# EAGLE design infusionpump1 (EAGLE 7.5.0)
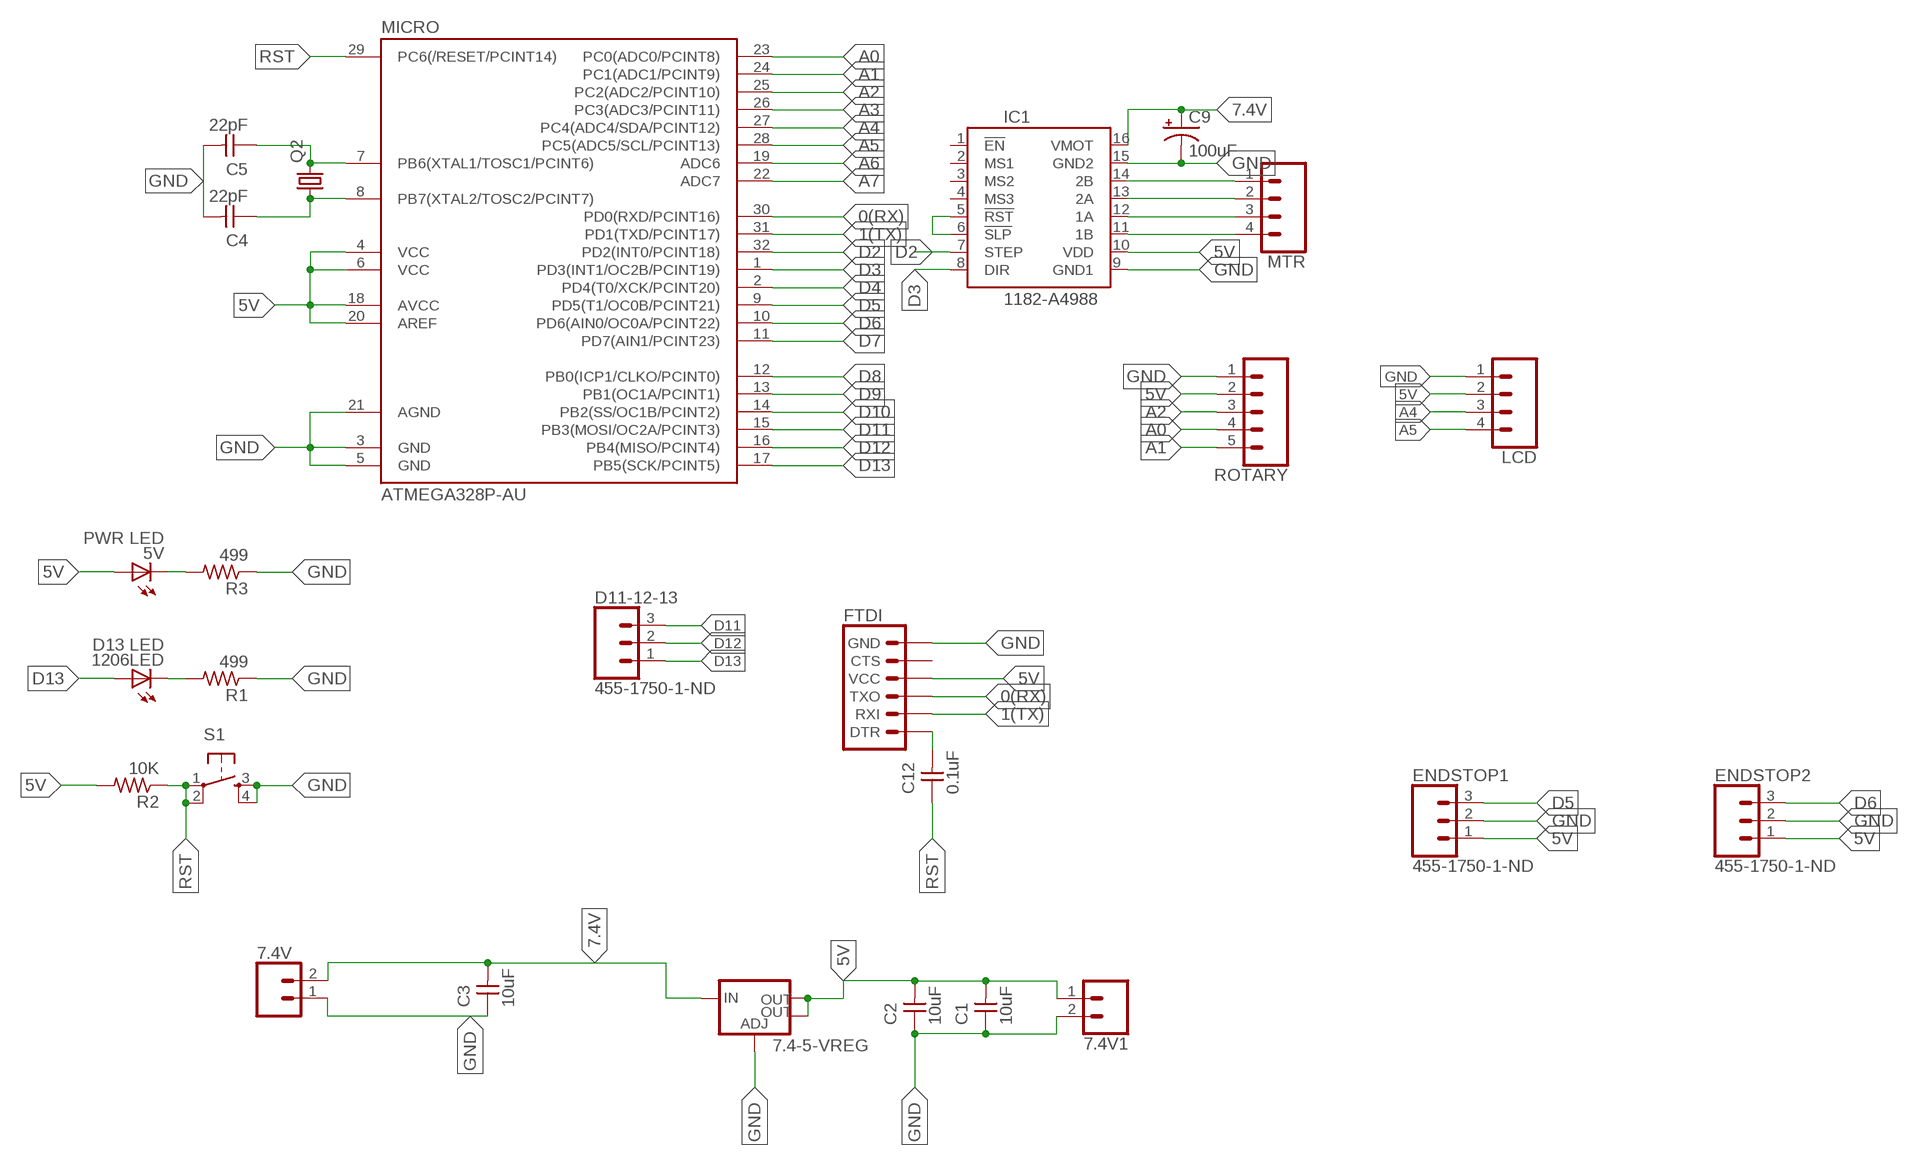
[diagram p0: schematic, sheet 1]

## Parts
5V  PWR LED  LEDFAB1206  [LED1206FAB]
7.4-5-VREG  V_REG_LM1117SOT223  [SOT223]
7.4V  CONN_02LOCK  [1X02_LOCK]
7.4V1  CONN_02LOCK  [1X02_LOCK]
1206LED  D13 LED  LEDFAB1206  [LED1206FAB]
C1  10uF  CAP-UNPOLARIZEDFAB  [C1206FAB]
C2  10uF  CAP-UNPOLARIZEDFAB  [C1206FAB]
C3  10uF  CAP-UNPOLARIZEDFAB  [C1206FAB]
C4  22pF  CAP-UNPOLARIZEDFAB  [C1206FAB]
C5  22pF  CAP-UNPOLARIZEDFAB  [C1206FAB]
C9  100uF  1000UF-RADIAL-5MM-25V-20%  [CPOL-RADIAL-5MM-10MM]
C12  0.1uF  CAP-UNPOLARIZEDFAB  [C1206FAB]
D11-12-13  455-1750-1-ND  CONN_03  [1X03]
ENDSTOP1  455-1750-1-ND  CONN_03  [1X03]
ENDSTOP2  455-1750-1-ND  CONN_03  [1X03]
FTDI  6_PIN_SERIAL_TARGET_SILK  [1X06]
IC1  1182-A4988  [A4988]
LCD  CONN_04  [1X04]
MICRO  ATMEGA328P-AU  ATMEGA48/88/168-AU  [TQFP32-08]
MTR  CONN_04  [1X04]
Q2  CRYSTALHC49U70  [HC49U70]
R1  499  RES-US1206FAB  [R1206FAB]
R2  10K  RES-US1206FAB  [R1206FAB]
R3  499  RES-US1206FAB  [R1206FAB]
ROTARY  CONN_05  [1X05]
S1  6MM_SWITCH6MM_SWITCH  [6MM_SWITCH]

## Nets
0(RX): FTDI.3(TXO) MICRO.30(PD0(RXD/PCINT16))
1(TX): FTDI.2(RXI) MICRO.31(PD1(TXD/PCINT17))
5V: 5V.1(A) 7.4-5-VREG.2(OUT) 7.4-5-VREG.4(OUT) 7.4V1.1 C1.2 C2.2 ENDSTOP1.1 ENDSTOP2.1 FTDI.4(VCC) IC1.10(VDD) LCD.2 MICRO.4(VCC) MICRO.6(VCC) MICRO.18(AVCC) MICRO.20(AREF) R2.2 ROTARY.2
7.4V: 7.4-5-VREG.3(IN) 7.4V.2 C3.2 C9.+ IC1.16(VMOT)
A0: MICRO.23(PC0(ADC0/PCINT8)) ROTARY.4
A1: MICRO.24(PC1(ADC1/PCINT9)) ROTARY.5
A2: MICRO.25(PC2(ADC2/PCINT10)) ROTARY.3
A3: MICRO.26(PC3(ADC3/PCINT11))
A4: LCD.3 MICRO.27(PC4(ADC4/SDA/PCINT12))
A5: LCD.4 MICRO.28(PC5(ADC5/SCL/PCINT13))
A6: MICRO.19(ADC6)
A7: MICRO.22(ADC7)
D2: IC1.7(STEP) MICRO.32(PD2(INT0/PCINT18))
D3: IC1.8(DIR) MICRO.1(PD3(INT1/OC2B/PCINT19))
D4: MICRO.2(PD4(T0/XCK/PCINT20))
D5: ENDSTOP1.3 MICRO.9(PD5(T1/OC0B/PCINT21))
D6: ENDSTOP2.3 MICRO.10(PD6(AIN0/OC0A/PCINT22))
D7: MICRO.11(PD7(AIN1/PCINT23))
D8: MICRO.12(PB0(ICP1/CLKO/PCINT0))
D9: MICRO.13(PB1(OC1A/PCINT1))
D10: MICRO.14(PB2(SS/OC1B/PCINT2))
D11: D11-12-13.3 MICRO.15(PB3(MOSI/OC2A/PCINT3))
D12: D11-12-13.2 MICRO.16(PB4(MISO/PCINT4))
D13: 1206LED.1(A) D11-12-13.1 MICRO.17(PB5(SCK/PCINT5))
GND: 7.4-5-VREG.1(ADJ) 7.4V1.2 7.4V.1 C1.1 C2.1 C3.1 C4.2 C5.2 C9.- ENDSTOP1.2 ENDSTOP2.2 FTDI.6(GND) IC1.5(!RST) IC1.6(!SLP) IC1.9(GND1) IC1.15(GND2) LCD.1 MICRO.3(GND) MICRO.5(GND) MICRO.21(AGND) R1.1 R3.1 ROTARY.1 S1.3(S) S1.4(S1)
N$1: 1206LED.2(C) R1.2
N$2: 5V.2(C) R3.2
N$3: C5.1 MICRO.7(PB6(XTAL1/TOSC1/PCINT6)) Q2.2
N$4: C4.1 MICRO.8(PB7(XTAL2/TOSC2/PCINT7)) Q2.1
N$6: IC1.14(2B) MTR.1
N$7: IC1.13(2A) MTR.2
N$8: IC1.12(1A) MTR.3
N$9: IC1.11(1B) MTR.4
N$16: C12.2 FTDI.1(DTR)
RST: C12.1 MICRO.29(PC6(/RESET/PCINT14)) R2.1 S1.1(P) S1.2(P1)
Unconnected: FTDI.5(CTS) IC1.1(!EN) IC1.2(MS1) IC1.3(MS2) IC1.4(MS3)

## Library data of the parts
5V 1206LED = fab:LED: LED
7.4-5-VREG = fab:V_REG_LM1117: Voltage Regulator LM1117 Standard adjustable voltage regulator but in SMD form. Spark Fun Electronics SKU : COM-00595; PROD_ID: VREG-08170
7.4V 7.4V1 = SparkFun-Connectors:CONN_02: Multi connection point. Often used as Generic Header-pin footprint for 0.1 inch spaced/style header connections
C1-C5 C12 = fab:CAP-UNPOLARIZED
C9 = SparkFun-Capacitors:1000UF: 1,000µF/1mF ceramic capacitors; PROD_ID: CAP-09538; VALUE: 1mF
D11-12-13 ENDSTOP1 ENDSTOP2 = SparkFun-Connectors:CONN_03: Multi connection point. Often used as Generic Header-pin footprint for 0.1 inch spaced/style header connections On any of the 0.1 inch spaced packages, you can populate with these: Break Away Headers - Straight (PRT-00116) Break Away Male Headers - Right Angle (PRT-00553) Female Headers (PRT-00115)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; PROD_ID: XXX-00000
FTDI = SparkFun-Connectors:6_PIN_SERIAL_TARGET: 6-pin header connection for use with the "FTDI BASIC" pinout - TARGET SIDE. Also known as "Arduino Serial Program Header". It is used to mate with our FTDI Basic serial programmers using the Arduino IDE. Note, this device has "TARGET" in the name. It is intended to be used on a design that contains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
IC1 = pololu-stepper-driver:1182-A4988: A4988 Stepper Motor Driver Carrier #1182 A4988 Stepper Motor Driver Carrier in Japan, Suzaku Lab. Ltd. #1182 A4988ステッピングモータドライバ
LCD MTR = SparkFun-Connectors:CONN_04: Multi connection point. Often used as Generic Header-pin footprint for 0.1 inch spaced/style header connections On any of the 0.1 inch spaced packages, you can populate with these: Break Away Headers - Straight (PRT-00116) Break Away Male Headers - Right Angle (PRT-00553) Female Headers (PRT-00115)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; PROD_ID: CONN-09696
MICRO = atmega8:ATMEGA48/88/168
Q2 = crystal:CRYSTAL: CRYSTAL; OC_FARNELL: unknown; OC_NEWARK: unknown
R1-R3 = fab:RES-US: Resistor (US Symbol)
ROTARY = SparkFun-Connectors:CONN_05: Multi connection point. Often used as Generic Header-pin footprint for 0.1 inch spaced/style header connections On any of the 0.1 inch spaced packages, you can populate with these: Break Away Headers - Straight (PRT-00116) Break Away Male Headers - Right Angle (PRT-00553) Female Headers (PRT-00115)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
S1 = fab:6MM_SWITCH: OMRON SWITCH

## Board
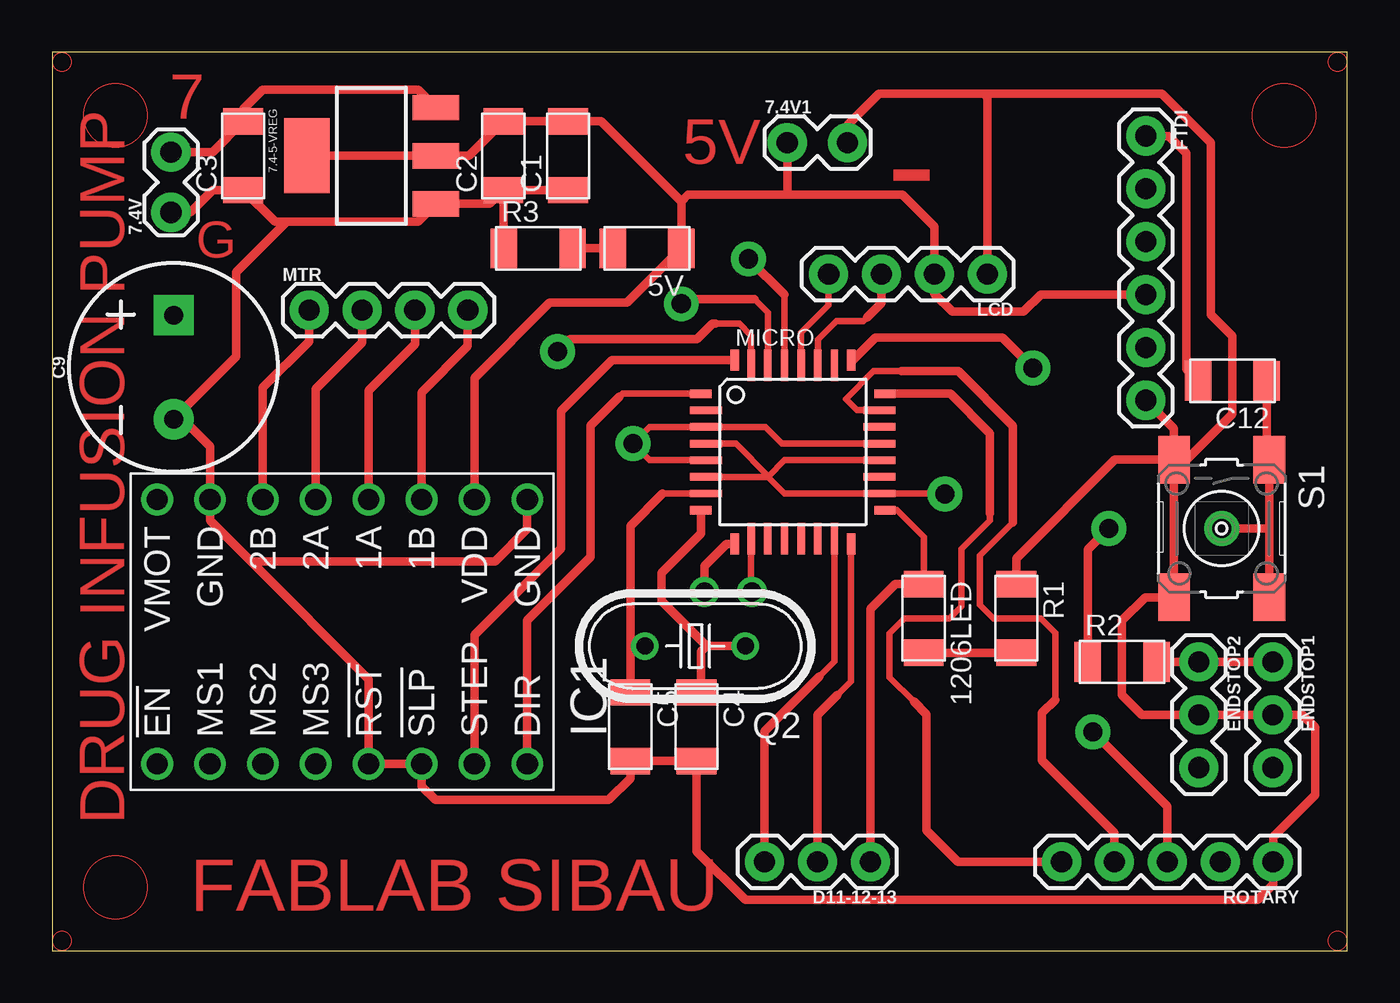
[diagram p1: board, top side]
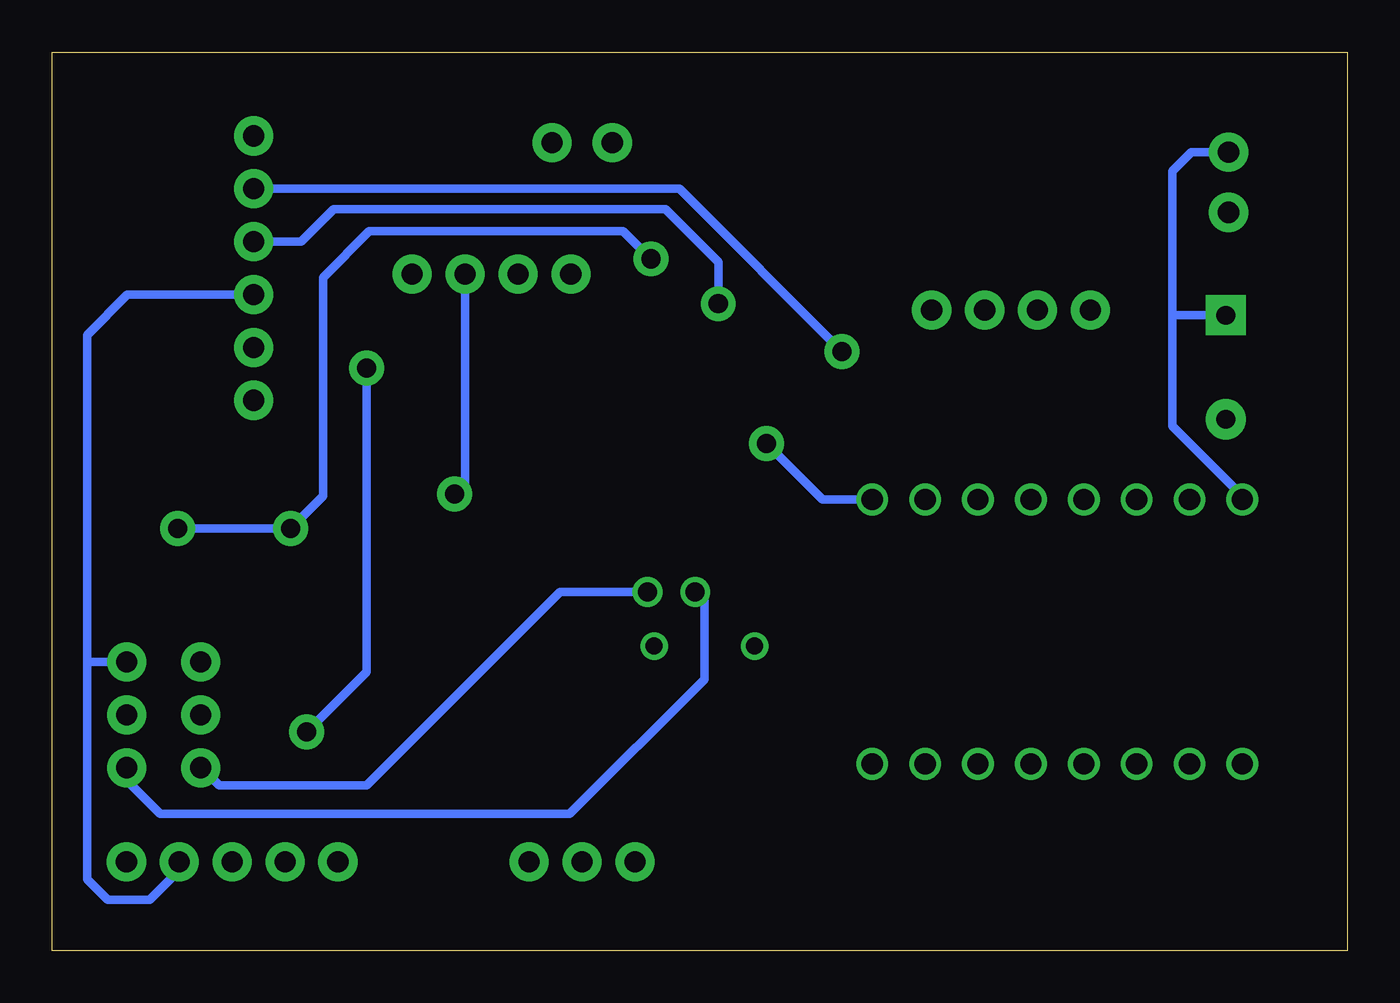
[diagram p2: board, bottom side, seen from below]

Size 62.23 x 43.18 mm. Coordinates in mm from the lower left corner, seen from the top.
Outline: 0,0 62.23,0 62.23,43.18 0,43.18 0,0
Copper layers (1*16): Top 0.035mm / dielectric 1.5mm / Bottom 0.035mm
Design rules "default *": minimum track width 10mil, minimum drill 24mil, track to track 12mil, track to pad 12mil, pad to pad 12mil, via to via 12mil, smd to smd 12mil, copper to edge 40mil, drill to drill 8mil, minimum pad ring 10mil, minimum via ring 8mil, stop-mask expansion 4mil, vias tented up to drill 0mil, thermal gap 10mil

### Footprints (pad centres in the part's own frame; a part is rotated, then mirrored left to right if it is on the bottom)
LED1206FAB = smd 1.27 x 1.905: 1 -1.651,0; 2 1.651,0
SOT223 = smd 1.219 x 2.235: 1 -2.311,-3.099; 2 0,-3.099; 3 2.311,-3.099 | smd 3.6 x 2.2: 4 0,3.099
1X02_LOCK = drill 1.016 pad 1.88: 1 -0.178,0; 2 2.718,0
C1206FAB = smd 1.27 x 1.905: 1 -1.651,0; 2 1.651,0
CPOL-RADIAL-5MM-10MM = drill 0.9 pad 1.93 square: + 2.5,0 | drill 0.9 pad 1.93: - -2.5,0
1X03 = drill 1.016 pad 1.88: 1 0,0; 2 2.54,0; 3 5.08,0
1X06 = drill 1.016 pad 1.88: 1 0,0; 2 2.54,0; 3 5.08,0; 4 7.62,0; 5 10.16,0; 6 12.7,0
A4988 = drill 1.016: 1 -6.35,8.89; 2 -6.35,6.35; 3 -6.35,3.81; 4 -6.35,1.27; 5 -6.35,-1.27; 6 -6.35,-3.81; 7 -6.35,-6.35; 8 -6.35,-8.89; 9 6.35,-8.89; 10 6.35,-6.35; 11 6.35,-3.81; 12 6.35,-1.27; 13 6.35,1.27; 14 6.35,3.81; 15 6.35,6.35; 16 6.35,8.89
1X04 = drill 1.016 pad 1.88: 1 0,0; 2 2.54,0; 3 5.08,0; 4 7.62,0
TQFP32-08 = smd 1.016 x 0.406: 1 -4.42,2.8; 8 -4.42,-2.8; 17 4.42,-2.8; 24 4.42,2.8 | smd 1.524 x 0.356: 2 -4.166,2; 3 -4.166,1.2; 4 -4.166,0.4; 5 -4.166,-0.4; 6 -4.166,-1.2; 7 -4.166,-2; 18 4.166,-2; 19 4.166,-1.2; 20 4.166,-0.4; 21 4.166,0.4; 22 4.166,1.2; 23 4.166,2 | smd 0.406 x 1.016: 9 -2.8,-4.42; 16 2.8,-4.42; 25 2.8,4.42; 32 -2.8,4.42 | smd 0.356 x 1.524: 10 -2,-4.166; 11 -1.2,-4.166; 12 -0.4,-4.166; 13 0.4,-4.166; 14 1.2,-4.166; 15 2,-4.166; 26 2,4.166; 27 1.2,4.166; 28 0.4,4.166; 29 -0.4,4.166; 30 -1.2,4.166; 31 -2,4.166
HC49U70 = drill 0.813: 1 -2.413,0; 2 2.413,0
R1206FAB = smd 1.27 x 1.905: 1 -1.651,0; 2 1.651,0
1X05 = drill 1.016 pad 1.88: 1 0,0; 2 2.54,0; 3 5.08,0; 4 7.62,0; 5 10.16,0
6MM_SWITCH = smd 2.286 x 1.524: 1 -3.302,2.286; 2 3.302,2.286; 3 -3.302,-2.286; 4 3.302,-2.286

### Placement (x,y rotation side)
5V  28.58,33.75 180 top
7.4-5-VREG  15.34,38.2 90 top
7.4V  5.71,35.66 90 top
7.4V1  35.5,38.83 0 top
1206LED  41.88,15.97 270 top
C1  24.78,38.2 90 top
C2  21.68,38.2 90 top
C3  9.18,38.2 90 top
C4  30.96,10.76 270 top
C5  27.78,10.76 270 top
C9  5.84,28.04 90 top
C12  56.7,27.39 180 top
D11-12-13  39.31,4.28 180 top
ENDSTOP1  58.64,13.88 270 top
ENDSTOP2  55.09,13.88 270 top
FTDI  52.55,39.15 270 top
IC1  13.94,15.34 90 top
LCD  44.93,32.51 180 top
MICRO  35.58,23.97 0 top
MTR  12.35,30.77 0 top
Q2  30.9,14.64 180 top
R1  46.32,15.97 270 top
R2  51.4,13.88 0 top
R3  23.35,33.75 0 top
ROTARY  58.66,4.28 180 top
S1  56.18,20.29 270 top

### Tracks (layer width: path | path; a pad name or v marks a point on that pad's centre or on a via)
0(RX)  (via drill 0.91 pad 1.68)
  Top 0.305: MICRO.30 34.38,30.67 33.75,31.3
  Top 0.406: 33.75,31.3 30.45,31.3 v30.23,31.08
  Bottom 0.406: FTDI.3 50.26,34.07 48.7,35.62 32.77,35.62 30.23,33.08 v30.23,31.08
1(TX)  (via drill 0.91 pad 1.68)
  Top 0.305: MICRO.31 33.59,29.57 33.02,30.13 31.88,30.13
  Top 0.406: 31.88,30.13 31.72,30.13 30.99,29.4 24.89,29.4 v24.29,28.8
  Bottom 0.406: FTDI.2 32.1,36.61 v24.29,28.8
5V  (via drill 0.91 pad 1.68)
  Top 0.305: 34.42,22.8 35.19,23.57 MICRO.20 | 34.42,22.8 34.39,22.77 | MICRO.6 34.39,22.77 | 34.39,22.77 35.19,21.97 MICRO.18 42.87,21.97 v42.89,21.94 | MICRO.4 32.85,24.37 34.42,22.8
  Top 0.406: 7.4-5-VREG.4 7.4-5-VREG.2 20.03,38.2 C2.2 C1.2 26.38,39.85 30.23,36 | FTDI.4 47.5,31.53 46.67,30.7 43.24,30.7 42.39,31.56 LCD.2 42.39,34.8 40.86,36.32 35.34,36.32 | R2.2 ENDSTOP2.1 ENDSTOP1.1 | IC1.10 20.29,27.53 23.91,31.15 27.63,31.15 5V.1 30.23,36 | 35.34,36.32 30.56,36.32 30.23,36 | 7.4V1.1 35.32,36.34 35.34,36.32
  Bottom 0.406: LCD.2 42.39,22.45 v42.89,21.94 | ROTARY.2 56.12,3.86 57.53,2.44 59.56,2.44 60.55,3.43 60.55,13.97 | FTDI.4 58.61,31.53 60.55,29.59 60.55,13.97 | ENDSTOP1.1 60.45,13.88 60.55,13.97
7.4V
  Top 0.406: 7.4-5-VREG.3 17.58,41.37 10.13,41.37 9.18,40.42 C3.2 7.71,38.37 7.4V.2
  Bottom 0.406: IC1.16 5.05,21.84 8.41,25.21 8.41,30.64 | 8.41,30.64 8.41,37.45 7.49,38.37 7.4V.2 | C9.+ 8.31,30.54 8.41,30.64
A0
  Top 0.305: 48.2,12.06 48.2,15.27 47.5,15.97 45.21,15.97 44.58,16.61 44.58,18.99 46.16,20.57 | 40.8,27.84 39.47,27.84 38.13,26.51 38.68,25.97 MICRO.23
  Top 0.406: 40.8,27.84 43.53,27.84 46.16,25.21 46.16,20.57 | ROTARY.4 51.04,5.67 47.56,9.14 47.56,11.43 48.2,12.06
A1
  Top 0.305: 41.53,11.84 41.4,11.97 40.23,13.14 40.23,15.24 40.96,15.97 43.12,15.97 43.69,16.54 43.69,19.3 45.05,20.67 45.05,21.02
  Top 0.406: MICRO.24 43.15,26.77 45.05,24.86 45.05,21.02 | ROTARY.5 43.51,4.28 42.01,5.78 42.01,11.37 41.4,11.97
A2  (via drill 0.91 pad 1.68)
  Top 0.406: MICRO.25 38.48,28.39 39.56,29.46 45.66,29.46 v47.12,28 | ROTARY.3 53.58,6.94 v50.01,10.51
  Bottom 0.406: v47.12,28 47.12,13.4 v50.01,10.51
A4
  Top 0.305: MICRO.27 36.78,29.36 37.69,30.26 38.99,30.26 39.15,30.42 39.47,30.73
  Top 0.406: LCD.3 39.85,31.11 39.15,30.42
A5
  Top 0.305: MICRO.28 35.98,29.7 37.31,31.02 LCD.4
D2
  Top 0.406: IC1.7 20.29,15.18 24.45,19.34 24.45,25.94 26.89,28.39 MICRO.32
D3
  Top 0.305: MICRO.1 27.4,26.77 27.27,26.64
  Top 0.406: IC1.8 22.83,15.88 25.88,18.92 25.88,25.24 27.27,26.64
D5  (via drill 0.91 pad 1.42)
  Top 0.406: v31.34,17.24 31.34,18.48 32.41,19.55 MICRO.9
  Bottom 0.406: ENDSTOP1.3 58.64,8.19 57.02,6.57 37.37,6.57 30.89,13.05 30.89,16.8 v31.34,17.24
D6  (via drill 0.91 pad 1.42)
  Top 0.305: MICRO.10 33.59,17.28 v33.62,17.24
  Bottom 0.406: v33.62,17.24 37.81,17.24 47.12,7.94 54.2,7.94 55.06,8.8 ENDSTOP2.3
D11
  Top 0.305: MICRO.15 37.59,13.9 36.72,13.03
  Top 0.406: 36.86,13.18 36.72,13.03 34.23,10.54 D11-12-13.3
D12
  Top 0.305: MICRO.16 38.38,12.95 37.29,11.86
  Top 0.406: 37.72,12.29 37.29,11.86 36.77,11.34 D11-12-13.2
D13
  Top 0.305: 1206LED.1 41.88,19.88 40.59,21.17 MICRO.17
  Top 0.406: D11-12-13.1 39.31,16.41 40.51,17.62 1206LED.1
GND  (via drill 0.91 pad 1.68)
  Top 0.254: 39.77,24.38 MICRO.21
  Top 0.305: MICRO.21 35.07,24.37 34.27,25.17 MICRO.3 28.71,25.17 v27.91,24.37 28.71,23.57 MICRO.5
  Top 0.406: 11.27,35.02 17.58,35.02 7.4-5-VREG.1 21.02,35.88 C2.1 | C2.1 21.68,33.77 R3.1 | C2.1 C1.1 | IC1.9 22.83,20.26 21.27,18.7 9.56,18.7 | 9.56,18.7 7.59,20.67 IC1.15 7.59,24.23 6.28,25.54 C9.- 8.85,28.54 8.85,32.6 11.27,35.02 | 9.56,18.7 15.21,13.05 IC1.5 IC1.6 17.75,7.91 18.41,7.24 26.73,7.24 27.78,8.29 C5.2 C4.2 30.96,4.79 33.31,2.44 57.91,2.44 58.66,3.19 ROTARY.1 58.66,5.48 60.67,7.49 60.67,10.73 60.07,11.34 ENDSTOP1.2 ENDSTOP2.2 52.35,11.34 51.4,12.29 51.4,15.88 52.51,16.99 S1.4 S1.3 | S1.3 53.9,25.09 FTDI.6 | S1.3 54.52,23.59 56.71,25.78 56.71,29.53 55.66,30.57 55.66,38.83 53.31,41.18 44.77,41.18 | R1.1 46.32,18.86 51.05,23.59 S1.3 | 7.4V.1 6.65,35.48 7.71,36.54 C3.1 10.71,35.02 11.27,35.02 | 7.4V1.2 38.21,39.67 39.72,41.18 44.77,41.18 | LCD.1 44.93,41.02 44.77,41.18
  Bottom 0.406: IC1.9 25.23,21.68 v27.91,24.37
N$1
  Top 0.406: R1.2 1206LED.2
N$2
  Top 0.406: 5V.2 R3.2
N$3
  Top 0.305: MICRO.7 29.33,21.97 28.57,21.21
  Top 0.406: C5.1 27.78,14.7 | 27.78,14.7 27.78,20.41 29.33,21.97 | Q2.2 27.84,14.64 27.78,14.7
N$4
  Top 0.406: C4.1 31.16,12.62 31.16,14.37 31.43,14.64 | Q2.1 31.43,14.64 | 31.43,14.64 29.27,16.8 29.27,18.16 31.16,20.05 MICRO.8
N$6
  Top 0.406: IC1.14 10.13,27.05 12.35,29.27 MTR.1
N$7
  Top 0.406: IC1.13 12.67,26.99 14.89,29.21 MTR.2
N$8
  Top 0.406: IC1.12 15.21,26.92 17.43,29.15 MTR.3
N$9
  Top 0.406: IC1.11 17.75,26.83 19.97,29.05 MTR.4
N$16
  Top 0.406: FTDI.1 53.66,39.15 54.48,38.32 54.48,27.95 C12.2
RST  (via drill 0.91 pad 1.68)
  Top 0.305: MICRO.29 35.19,31.52
  Top 0.406: S1.2 58.47,20.19 | 58.47,20.19 58.47,22.95 | 58.47,22.95 S1.1 | C12.1 58.35,23.07 58.47,22.95 | R2.1 49.75,19.27 v50.77,20.29 | v33.47,33.24 35.19,31.52 | v56.19,20.29 58.38,20.29 58.47,20.19
  Bottom 0.406: v33.47,33.24 34.8,34.58 46.99,34.58 49.21,32.35 49.21,21.84 v50.77,20.29 v56.19,20.29
(copper drawn outside any net)
  shapes: Top circle x7

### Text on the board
Top: 7 | 5V | - | G | DRUG INFUSION PUMP | FABLAB SIBAU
